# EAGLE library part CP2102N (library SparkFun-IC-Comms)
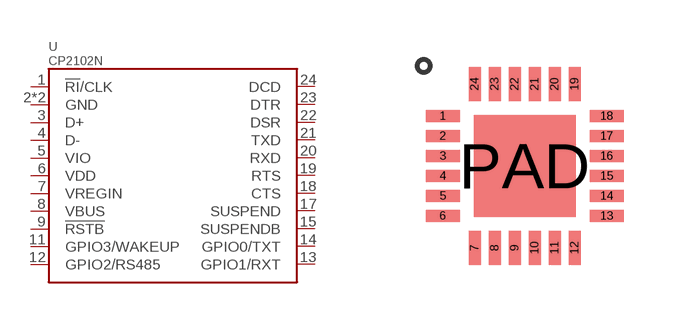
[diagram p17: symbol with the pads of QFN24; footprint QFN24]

Designator prefix U

## CP2102N (PROD_ID: IC-14020)  [QFN24]
1  !RI!/CLK
2  GND
3  D+
4  D-
5  VIO
6  VDD
7  VREGIN
8  VBUS
9  !RSTB
11  GPIO3/WAKEUP
12  GPIO2/RS485
13  GPIO1/RXT
14  GPIO0/TXT
15  SUSPENDB
17  SUSPEND
18  CTS
19  RTS
20  RXD
21  TXD
22  DSR
23  DTR
24  DCD
PAD  GND

## Footprint QFN24 (pad centres in mm)
smd 0.85 x 0.3: 1 -2.05,1.25; 2 -2.05,0.75; 3 -2.05,0.25; 4 -2.05,-0.25; 5 -2.05,-0.75; 6 -2.05,-1.25; 13 2.05,-1.25; 14 2.05,-0.75; 15 2.05,-0.25; 16 2.05,0.25; 17 2.05,0.75; 18 2.05,1.25
smd 0.3 x 0.85: 7 -1.25,-2.05; 8 -0.75,-2.05; 9 -0.25,-2.05; 10 0.25,-2.05; 11 0.75,-2.05; 12 1.25,-2.05; 19 1.25,2.05; 20 0.75,2.05; 21 0.25,2.05; 22 -0.25,2.05; 23 -0.75,2.05; 24 -1.25,2.05
smd 2.55 x 2.55: PAD 0,0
